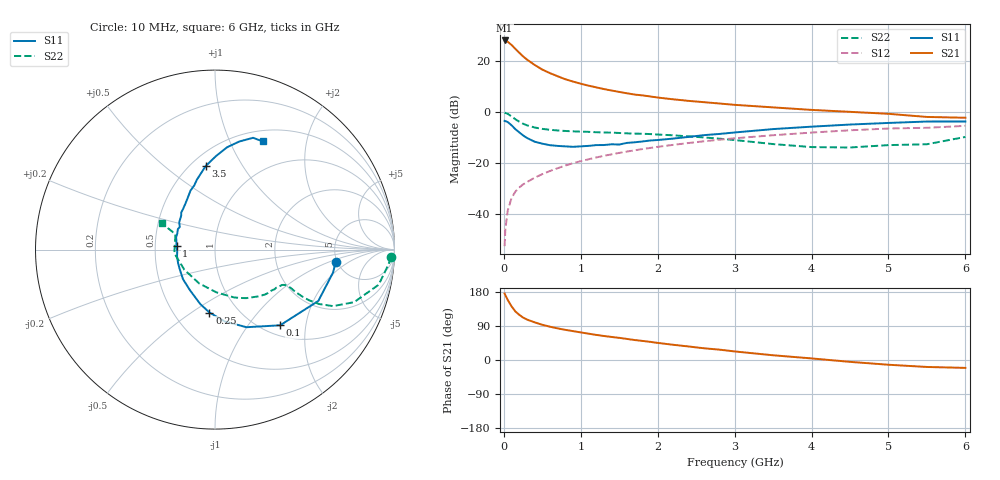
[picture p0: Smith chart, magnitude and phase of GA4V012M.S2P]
! Infineon Technologies  Discrete & RF Semiconductors
! BF775
! Si NPN RF Bipolar Junction Transistor in SOT23
! VCE = 4 V  IC = 12 mA
! Common Emitter S-Parameters:  May  1996
# GHz  S  MA  R  50
!  f  S11  S21  S12  S22
! GHz  MAG  ANG  MAG  ANG  MAG  ANG  MAG  ANG
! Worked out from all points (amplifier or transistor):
!   36 points, 10 MHz to 6 GHz, reference 50 ohm
!   highest |S21| = 28.1 dB at 10 MHz (marker M1)
!   |S21| within 3 dB of that: start of sweep to 140.3 MHz
!   unconditionally stable (mu >= 1): 524.4 MHz to 3.154 GHz
!   at 250 MHz: K = 0.73, MSG = 25.0 dB, |S12| = -28.2 dB
!   at 1.4 GHz: K = 1.10, MAG = 10.5 dB, |S12| = -16.5 dB
!   at 6 GHz: K = 0.94, MSG = 1.6 dB, |S12| = -5.3 dB
!   S11 on the Smith chart (normalised r, x): 10 MHz: 4.86, -1.20; 100 MHz: 1.18, -1.44; 250 MHz: 0.74, -0.59; 1 GHz: 0.65, +0.03; 3.5 GHz: 0.59, +0.70; 6 GHz: 0.63, +1.33
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0.01  0.6758 -5.7  25.35 175.4  0.0024 93.6  0.9822 -2.4
0.02  0.6703 -10.9  25.19 170.8  0.0052 81.3  0.9696 -5.0
0.05  0.6429 -26.4  23.97 158.8  0.0118 78.9  0.9327 -12.1
0.1  0.5563 -49.3  20.7 141.7  0.021 70.7  0.8286 -20.7
0.15  0.4667 -67.9  17.34 128.2  0.028 65.5  0.7288 -25.6
0.2  0.4042 -82.2  14.59 119.2  0.0336 64.3  0.6544 -27.6
0.25  0.352 -95.0  12.39 112.0  0.0388 62.9  0.5963 -28.3
0.3  0.3145 -105.1  10.74 106.8  0.0429 63.8  0.5559 -28.3
0.4  0.2655 -121.8  8.42 99.4  0.0524 64.2  0.5036 -27.7
0.5  0.2427 -137.3  6.827 92.9  0.0615 65.5  0.4723 -26.8
0.6  0.2265 -149.1  5.812 87.8  0.0709 66.3  0.4535 -26.8
0.8  0.215 -169.6  4.415 79.5  0.0908 66.5  0.4302 -27.2
1  0.2152 175.0  3.615 72.8  0.1105 66.1  0.4181 -28.7
1.1  0.2197 168.0  3.313 69.5  0.1201 65.6  0.4133 -29.6
1.3  0.2282 157.0  2.84 63.4  0.1404 64.3  0.4011 -32.1
1.6  0.2513 142.6  2.345 55.6  0.1701 61.9  0.3865 -36.7
2.2  0.305 122.7  1.791 40.2  0.23 56.1  0.3538 -47.6
3  0.4018 104.6  1.395 22.6  0.3092 46.9  0.286 -68.5
3.5  0.4682 96.4  1.244 12.5  0.355 40.6  0.2383 -88.1
4.5  0.5746 83.2  1.018 -4.9  0.4435 27.5  0.2043 -146.7
5.5  0.658 71.2  0.809 -18.4  0.4964 12.7  0.2365 158.7
6  0.6587 66.3  0.78 -20.8  0.5414 8.6  0.3289 153.7
